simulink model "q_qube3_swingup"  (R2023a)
settings: Solver=ode4  StartTime=0.0  StopTime=inf  FixedStep=0.002  RelTol=1e-3  EnableMultiTasking=on
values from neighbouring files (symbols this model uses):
  g = 9.81    [parameter.m]    (also in qube2_rotpen_param.m)
  Jp_cm = mp*lp^2/12    (= 3.3282e-05)    [parameter.m]
  K = lqr(A,B,Q_1,R)    [setup.m]
  kt = 0.0422    [parameter.m]    (also in qube2_rotpen_param.m = 0.042)
  lp = 0.129    [parameter.m]
  lr = 0.085    [parameter.m]
  mp = 0.024    [parameter.m]    (also in qube2_rotpen_param.m)
  mr = 0.095    [parameter.m]    (also in qube2_rotpen_param.m)
  Rm = 7.5    [parameter.m]    (also in qube2_rotpen_param.m = 8.4)
undefined symbols (not defined in the file or in its folder): HIL, qc_get_step_size
libraries: simulink x3, quarc_library x3, simulink_extras x3

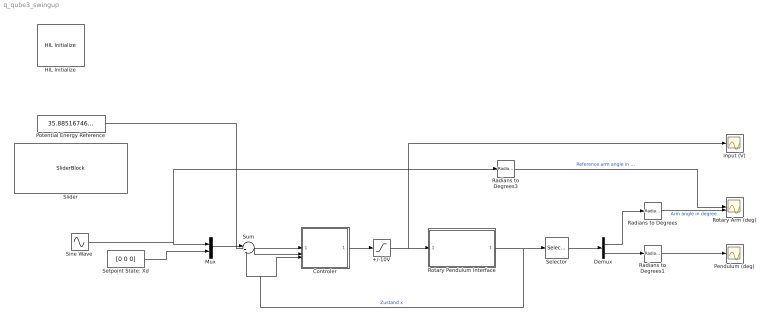
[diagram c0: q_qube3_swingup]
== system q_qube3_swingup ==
  +/-10V : Saturate  UpperLimit=10  LowerLimit=-10
  Controler : Subsystem
  Demux : Demux  Outputs=2
  HIL Initialize : quarc_library/Data Acquisition/Generic/Configuration/HIL Initialize  object_name=HIL-1  board_type=qube_servo3_usb  board_number=0  board_options=deadband_compensation=0.65;pwm_en=0;enc0_velocity=3.0;enc1_velocity=3.0;  exclusive=off  active=off  hardware_clocks=[0]  clock_modes=[]  initial_clock_frequencies=[]  set_clock_params_at_start=off  set_clock_params_at_switch_in=off  set_clock_frequencies_at_start=off  set_clock_frequencies_at_switch_in=off  analog_input_channels=[0]  analog_input_configurations=[]  analog_input_maximums=3  analog_input_minimums=-3  set_analog_input_params_at_start=off  set_analog_input_params_at_switch_in=off  analog_output_channels=[0]  analog_output_maximums=15  analog_output_minimums=-15  initial_analog_outputs=[0]  final_analog_outputs=[0]  watchdog_analog_outputs=0  set_analog_output_params_at_start=off  set_analog_output_params_at_switch_in=off  set_analog_outputs_at_start=on  set_analog_outputs_at_switch_in=off  set_analog_outputs_at_terminate=on  set_analog_outputs_at_switch_out=off  set_analog_outputs_on_watchdog=on  digital_input_channels=[]  digital_output_channels=[0]  digital_output_configuration=[]  initial_digital_outputs=[1]  final_digital_outputs=[0]  watchdog_digital_outputs=[0]  set_digital_output_params_at_start=off  set_digital_output_params_at_switch_in=off  set_digital_outputs_at_start=on  set_digital_outputs_at_switch_in=off  set_digital_outputs_at_terminate=on  set_digital_outputs_at_switch_out=off  set_digital_outputs_on_watchdog=on  encoder_channels=[0:1]  quadrature=[4]  encoder_filter_frequency=[]  initial_encoder_counts=[0]  set_encoder_params_at_start=off  set_encoder_params_at_switch_in=off  set_encoder_counts_at_start=on  set_encoder_counts_at_switch_in=off  pwm_channels=[]  pwm_modes=[0]  pwm_frequency=23195  pwm_configuration=[1]  pwm_alignment=[0]  pwm_polarity=[1]  pwm_leading_deadband=[0]  pwm_trailing_deadband=[0]  initial_pwm_outputs=[0]  final_pwm_outputs=[0]  watchdog_pwm_outputs=[]  set_pwm_params_at_start=off  set_pwm_params_at_switch_in=off  set_pwm_outputs_at_start=off  set_pwm_outputs_at_switch_in=off  set_pwm_outputs_at_terminate=off  set_pwm_outputs_at_switch_out=off  set_pwm_outputs_on_watchdog=off  other_output_channels=[11000:11002]  initial_other_outputs=[0 1 0]  final_other_outputs=[1 0 0]  watchdog_other_outputs=[0 0 1]  set_other_outputs_at_start=on  set_other_outputs_at_switch_in=off  set_other_outputs_at_terminate=on  set_other_outputs_at_switch_out=off  set_other_outputs_on_watchdog=on
  Input (V) : Scope
  Mux : Mux  Inputs=2
  Pendulum (deg) : Scope
  Potential Energy Reference : Constant  Value=35.88516746411483
  Radians to Degrees : simulink_extras/Transformations/Radians to Degrees
  Radians to Degrees1 : simulink_extras/Transformations/Radians to Degrees
  Radians to Degrees3 : simulink_extras/Transformations/Radians to Degrees
  Rotary Arm (deg) : Scope  NumInputPorts=2
  Rotary Pendulum Interface : Subsystem
  Selector : Selector  InputPortWidth=4  IndexOptions=Index vector (dialog)  Indices=[1 2]  OutputSizes=1
  Setpoint State: Xd : Constant  Value=[0 0 0]
  Sine Wave : Sin  SampleTime=0
  Slider : SliderBlock
  Sum : Sum  Inputs=|+-
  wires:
  Mux/1 -> Sum/1
  Radians to Degrees/1 -> Rotary Arm (deg)/2  "Arm angle in degree"
  Radians to Degrees1/1 -> Pendulum (deg)/1
  Rotary Pendulum Interface/1(X) -> Sum/2, Controler/3(x), Selector/1  "Zustand x"
  Selector/1 -> Demux/1
  Demux/1 -> Radians to Degrees/1
  Demux/2 -> Radians to Degrees1/1
  +/-10V/1 -> Input (V)/1, Rotary Pendulum Interface/1(u (V))
  Setpoint State: Xd/1 -> Mux/2
  Radians to Degrees3/1 -> Rotary Arm (deg)/1  "Reference arm angle in degree"
  Sine Wave/1 -> Radians to Degrees3/1, Mux/1
  Potential Energy Reference/1 -> Controler/1(Er (mJ))
  Sum/1 -> Controler/2(e)
  Controler/1(u'(V)) -> +/-10V/1

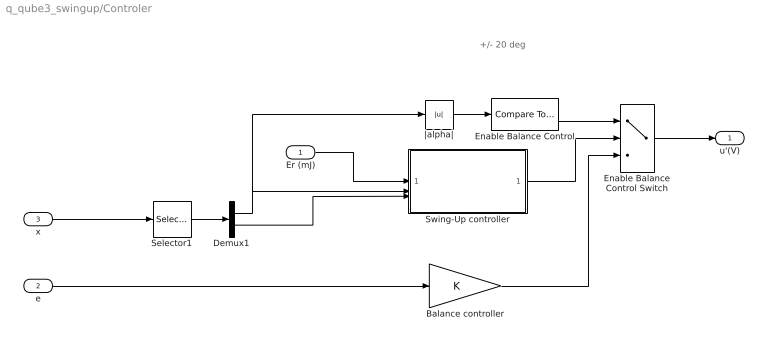
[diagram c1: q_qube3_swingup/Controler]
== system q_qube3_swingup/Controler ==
  note: +/- 20 deg
  Er (mJ) : Inport
  e : Inport  Port=2
  x : Inport  Port=3
  Balance controller : Gain  Gain=K  Multiplication=Matrix(K*u)
  Demux1 : Demux  Outputs=2
  Enable Balance Control : simulink/Logic and Bit Operations/Compare To Constant  relop=<=  const=20*pi/180  OutDataTypeStr=uint8  ZeroCross=off
  Enable Balance Control Switch : MultiPortSwitch  DataPortOrder=Zero-based contiguous  Inputs=2  zeroidx=on
  Selector1 : Selector  InputPortWidth=4  IndexOptions=Index vector (dialog)  Indices=[2,4]  OutputSizes=1
  Swing-Up controller : Subsystem
  |alpha| : Abs
  u'(V) : Outport
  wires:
  |alpha|/1 -> Enable Balance Control/1
  Balance controller/1 -> Enable Balance Control Switch/3
  Enable Balance Control Switch/1 -> u'(V)/1
  Demux1/1 -> |alpha|/1, Swing-Up controller/2(In2)
  Enable Balance Control/1 -> Enable Balance Control Switch/1
  Selector1/1 -> Demux1/1
  e/1 -> Balance controller/1
  Er (mJ)/1 -> Swing-Up controller/1(Er (mJ))
  Demux1/2 -> Swing-Up controller/3(alpha_dot (rad/s))
  Swing-Up controller/1(Out1) -> Enable Balance Control Switch/2
  x/1 -> Selector1/1

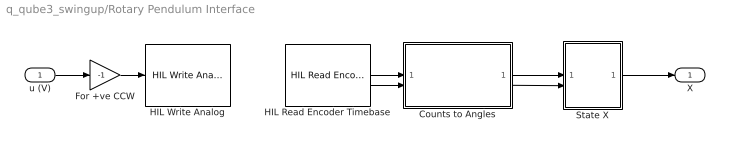
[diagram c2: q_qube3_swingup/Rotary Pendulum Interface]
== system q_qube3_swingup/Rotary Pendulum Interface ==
  u (V) : Inport
  Counts to Angles : Subsystem
  For +ve CCW : Gain  Gain=-1
  HIL Read Encoder Timebase : quarc_library/Data Acquisition/Generic/Timebases/HIL Read Encoder Timebase  object_name=HIL-1  clock=0  channels=[0:1]  active=on  vector_output=off  data_type_mode=Inherit via back propagation  data_type=double  overflow_mode=Error on overflow  samples_in_buffer=max(ceil(1/qc_get_step_size), 1)
  HIL Write Analog : quarc_library/Data Acquisition/Generic/Immediate I//O/HIL Write Analog  object_name=HIL-1  channels=0  sample_time=-1  active=off  vector_input=off
  State X : Subsystem
  X : Outport  VectorParamsAs1DForOutWhenUnconnected=off
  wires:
  For +ve CCW/1 -> HIL Write Analog/1
  Counts to Angles/2(alpha (rad)) -> State X/2(alpha)
  Counts to Angles/1(theta (rad)) -> State X/1(theta)
  State X/1(X) -> X/1
  u (V)/1 -> For +ve CCW/1
  HIL Read Encoder Timebase/1 -> Counts to Angles/1(arm enc)
  HIL Read Encoder Timebase/2 -> Counts to Angles/2(pen enc)

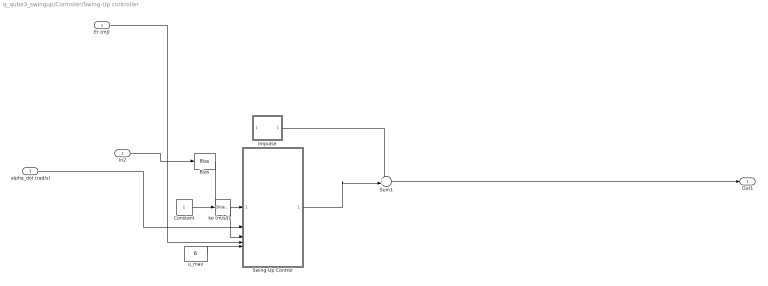
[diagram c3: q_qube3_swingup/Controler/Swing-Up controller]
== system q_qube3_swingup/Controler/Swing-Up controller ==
  Er (mJ) : Inport
  In2 : Inport  Port=2
  alpha_dot (rad/s) : Inport  Port=3
  Bias : Bias  Bias=+pi
  Constant : Constant
  Impulse : Subsystem
  Sum1 : Sum  Inputs=++|
  Swing-Up Control : Subsystem
  ke (m/s/J) : simulink/Math Operations/Slider Gain  gain=36.0  low=0  high=100
  u_max : Constant  Value=6
  Out1 : Outport
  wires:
  In2/1 -> Bias/1
  u_max/1 -> Swing-Up Control/5(u_max (m/s^2))
  Er (mJ)/1 -> Swing-Up Control/4(Er (mJ))
  Swing-Up Control/1(u (V)) -> Sum1/2
  ke (m/s/J)/1 -> Swing-Up Control/3(ke (m/s/J))
  Bias/1 -> Swing-Up Control/1(alpha_f (rad))
  Impulse/1(u (V)) -> Sum1/1
  Constant/1 -> ke (m/s/J)/1
  alpha_dot (rad/s)/1 -> Swing-Up Control/2(alpha_dot (rad/s))
  Sum1/1 -> Out1/1

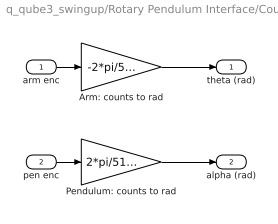
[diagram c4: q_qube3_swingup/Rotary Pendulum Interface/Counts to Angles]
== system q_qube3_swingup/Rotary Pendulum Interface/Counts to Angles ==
  arm enc : Inport
  pen enc : Inport  Port=2
  Arm: counts to rad : Gain  Gain=-2*pi/512/4
  Pendulum: counts to rad : Gain  Gain=2*pi/512/4
  theta (rad) : Outport  VectorParamsAs1DForOutWhenUnconnected=off
  alpha (rad) : Outport  Port=2  VectorParamsAs1DForOutWhenUnconnected=off
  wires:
  pen enc/1 -> Pendulum: counts to rad/1
  arm enc/1 -> Arm: counts to rad/1
  Arm: counts to rad/1 -> theta (rad)/1
  Pendulum: counts to rad/1 -> alpha (rad)/1

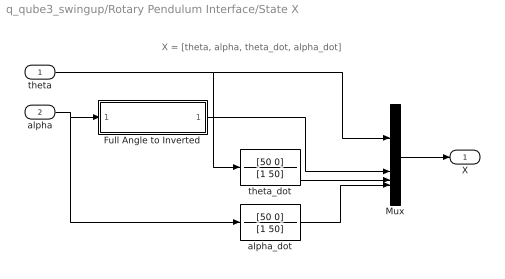
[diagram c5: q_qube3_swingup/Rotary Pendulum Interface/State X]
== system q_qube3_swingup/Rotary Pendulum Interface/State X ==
  note: X = [theta, alpha, theta_dot, alpha_dot]
  theta : Inport
  alpha : Inport  Port=2
  Full Angle to Inverted : Subsystem
  Mux : Mux
  alpha_dot : TransferFcn  Numerator=[50 0]  Denominator=[1 50]
  theta_dot : TransferFcn  Numerator=[50 0]  Denominator=[1 50]
  X : Outport  VectorParamsAs1DForOutWhenUnconnected=off
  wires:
  Mux/1 -> X/1
  alpha/1 -> alpha_dot/1, Full Angle to Inverted/1(alpha (rad))
  theta/1 -> theta_dot/1, Mux/1
  theta_dot/1 -> Mux/3
  alpha_dot/1 -> Mux/4
  Full Angle to Inverted/1(alpha_up) -> Mux/2

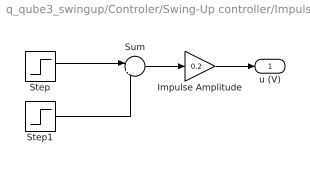
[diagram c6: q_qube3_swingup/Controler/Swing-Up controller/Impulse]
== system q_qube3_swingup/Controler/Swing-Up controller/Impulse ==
  Impulse Amplitude : Gain  Gain=0.2
  Step : Step  SampleTime=0
  Step1 : Step  Time=1.1  After=-1  SampleTime=0
  Sum : Sum  Inputs=|++
  u (V) : Outport  VectorParamsAs1DForOutWhenUnconnected=off
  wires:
  Step1/1 -> Sum/2
  Step/1 -> Sum/1
  Sum/1 -> Impulse Amplitude/1
  Impulse Amplitude/1 -> u (V)/1

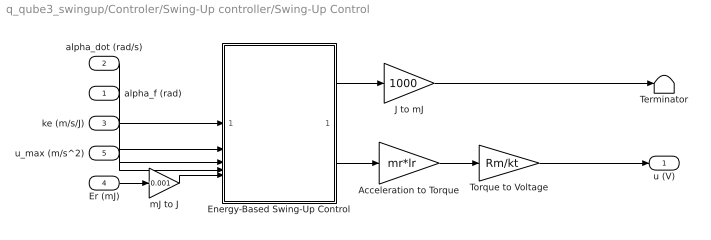
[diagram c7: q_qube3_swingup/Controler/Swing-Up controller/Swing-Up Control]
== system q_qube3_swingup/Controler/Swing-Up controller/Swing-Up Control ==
  alpha_f (rad) : Inport
  alpha_dot (rad/s) : Inport  Port=2
  ke (m/s/J) : Inport  Port=3
  Er (mJ) : Inport  Port=4
  u_max (m/s^2) : Inport  Port=5
  Acceleration to Torque : Gain  Gain=mr*lr
  Energy-Based Swing-Up Control : Subsystem
  J to mJ : Gain  Gain=1000
  Terminator : Terminator
  Torque to Voltage : Gain  Gain=Rm/kt
  mJ to J : Gain  Gain=0.001
  u (V) : Outport  VectorParamsAs1DForOutWhenUnconnected=off
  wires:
  Energy-Based Swing-Up Control/2(u (m/s^2)) -> Acceleration to Torque/1
  Energy-Based Swing-Up Control/1(E (J)) -> J to mJ/1
  alpha_f (rad)/1 -> Energy-Based Swing-Up Control/2(a_f (rad))
  ke (m/s/J)/1 -> Energy-Based Swing-Up Control/3(ke (m/s/J))
  u_max (m/s^2)/1 -> Energy-Based Swing-Up Control/4(u_max (m/s^2))
  Acceleration to Torque/1 -> Torque to Voltage/1
  Er (mJ)/1 -> mJ to J/1
  J to mJ/1 -> Terminator/1
  Torque to Voltage/1 -> u (V)/1
  alpha_dot (rad/s)/1 -> Energy-Based Swing-Up Control/1(a_dot (rad/s))
  mJ to J/1 -> Energy-Based Swing-Up Control/5(Er (J))

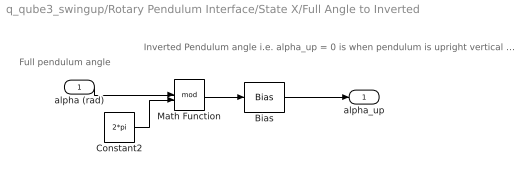
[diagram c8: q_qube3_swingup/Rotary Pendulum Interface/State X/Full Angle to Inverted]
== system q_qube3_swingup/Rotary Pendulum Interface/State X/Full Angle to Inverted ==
  note: Inverted Pendulum angle i.e. alpha_up = 0 is when pendulum is upright vertical position
  note: Full pendulum angle
  alpha (rad) : Inport
  Bias : Bias  Bias=-pi
  Constant2 : Constant  Value=2*pi
  Math Function : Math  Operator=mod  SignedPower=on
  alpha_up : Outport  VectorParamsAs1DForOutWhenUnconnected=off
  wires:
  Constant2/1 -> Math Function/2
  alpha (rad)/1 -> Math Function/1
  Bias/1 -> alpha_up/1
  Math Function/1 -> Bias/1

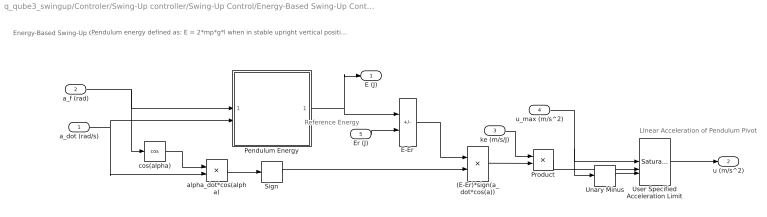
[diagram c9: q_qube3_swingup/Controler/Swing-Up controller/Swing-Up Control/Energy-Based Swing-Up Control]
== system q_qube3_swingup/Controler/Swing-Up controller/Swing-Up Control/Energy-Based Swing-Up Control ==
  note: Energy-Based Swing-Up Control
  note: LInear Acceleration of Pendulum Pivot
  note: Reference Energy
  note: Pendulum energy defined as: E = 2*mp*g*l when in stable upright vertical position E = 0 when in downward position
  a_dot (rad/s) : Inport
  a_f (rad) : Inport  Port=2
  ke (m/s/J) : Inport  Port=3
  u_max (m/s^2) : Inport  Port=4
  Er (J) : Inport  Port=5
  (E-Er)*sign(a_dot*cos(a)) : Product  RndMeth=Zero
  E-Er : Sum  Inputs=+-
  Pendulum Energy : Subsystem
  Product : Product  RndMeth=Zero
  Sign : Signum
  Unary Minus : UnaryMinus
  User Specified Acceleration Limit : simulink/Discontinuities/Saturation Dynamic  OutMin=[]  OutMax=[]  OutDataTypeStr=Inherit: Same as second input  OutDataType=fixdt(1, 16)  OutScaling=2^-10  DoSatur=off
  alpha_dot*cos(alpha) : Product  RndMeth=Zero
  cos(alpha) : Trigonometry  Operator=cos
  E (J) : Outport  VectorParamsAs1DForOutWhenUnconnected=off
  u (m/s^2) : Outport  Port=2  VectorParamsAs1DForOutWhenUnconnected=off
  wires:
  a_f (rad)/1 -> Pendulum Energy/1(alpha (rad)), cos(alpha)/1
  Sign/1 -> (E-Er)*sign(a_dot*cos(a))/2
  alpha_dot*cos(alpha)/1 -> Sign/1
  cos(alpha)/1 -> alpha_dot*cos(alpha)/1
  E-Er/1 -> (E-Er)*sign(a_dot*cos(a))/1
  Pendulum Energy/1(E (J)) -> E (J)/1, E-Er/1
  a_dot (rad/s)/1 -> alpha_dot*cos(alpha)/2, Pendulum Energy/2(alpha_dot (rad/s))
  (E-Er)*sign(a_dot*cos(a))/1 -> Product/2
  Er (J)/1 -> E-Er/2
  ke (m/s/J)/1 -> Product/1
  Product/1 -> User Specified Acceleration Limit/2
  u_max (m/s^2)/1 -> User Specified Acceleration Limit/1, Unary Minus/1
  Unary Minus/1 -> User Specified Acceleration Limit/3
  User Specified Acceleration Limit/1 -> u (m/s^2)/1

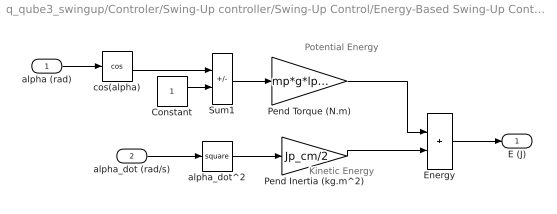
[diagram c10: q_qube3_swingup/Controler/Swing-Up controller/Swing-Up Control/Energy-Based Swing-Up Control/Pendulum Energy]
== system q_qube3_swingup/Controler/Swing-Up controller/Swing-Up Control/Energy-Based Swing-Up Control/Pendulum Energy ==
  note: Kinetic Energy
  note: Potential Energy
  alpha (rad) : Inport
  alpha_dot (rad/s) : Inport  Port=2
  Constant : Constant
  Energy : Sum  SaturateOnIntegerOverflow=on
  Pend Inertia (kg.m^2) : Gain  Gain=Jp_cm/2
  Pend Torque (N.m) : Gain  Gain=mp*g*lp/2
  Sum1 : Sum  Inputs=-+  SaturateOnIntegerOverflow=on
  alpha_dot^2 : Math  Operator=square  SignedPower=on
  cos(alpha) : Trigonometry  Operator=cos
  E (J) : Outport  VectorParamsAs1DForOutWhenUnconnected=off
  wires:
  Sum1/1 -> Pend Torque (N.m)/1
  Constant/1 -> Sum1/2
  Pend Inertia (kg.m^2)/1 -> Energy/2
  alpha_dot^2/1 -> Pend Inertia (kg.m^2)/1
  Pend Torque (N.m)/1 -> Energy/1
  alpha (rad)/1 -> cos(alpha)/1
  alpha_dot (rad/s)/1 -> alpha_dot^2/1
  Energy/1 -> E (J)/1
  cos(alpha)/1 -> Sum1/1
